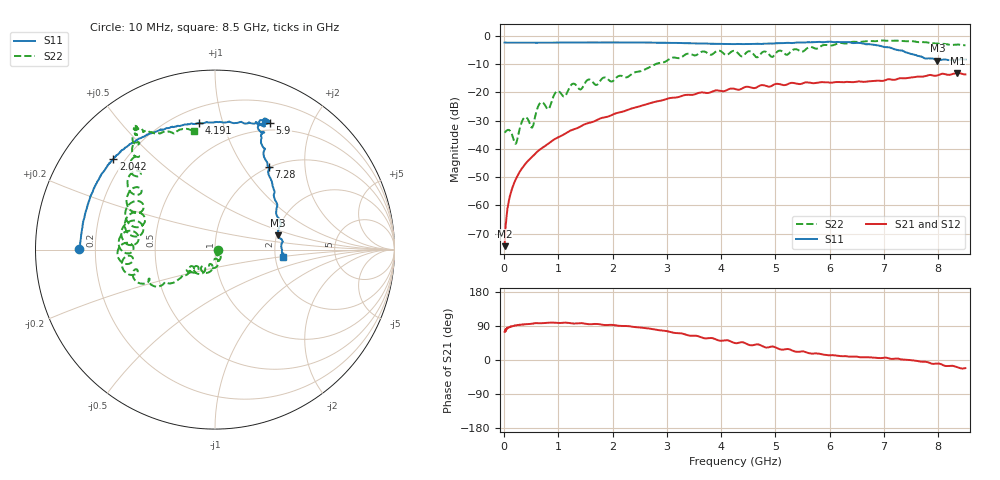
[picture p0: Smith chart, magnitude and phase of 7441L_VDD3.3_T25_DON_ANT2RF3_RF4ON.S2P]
!Agilent Technologies,E5071C,MY46417908,A.11.23
!Date: Mon May 03 19:54:48 2021
!Data & Calibration Information:
!Freq	S11:SOLT2(ON)	S21:SOLT2(ON)	S12:SOLT2(ON)	S22:SOLT2(ON)
!PortZ  Port1:50+j0  Port2:50+j0
!Above PortZ is port z conversion or system Z0 setting when saving the data.
!When reading, reference impedance value at option line is always used.
# Hz S dB R 50
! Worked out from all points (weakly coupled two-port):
!   1601 points, 10 MHz to 8.5 GHz, reference 50 ohm
!   highest |S21| = -13.24 dB at 8.351 GHz (marker M1); lowest = -74.4 dB at 10 MHz (marker M2)
!   lowest |S11| = -8.9 dB at 7.985 GHz (marker M3), VSWR 2.13, Z = 102 + j18.6 ohm
!   |S11| at or under -10 dB: nowhere
!   |S22| runs from -38.2 to -1.7 dB; largest |S21 - S12| = 0.0021
!   S11 on the Smith chart (normalised r, x): 10 MHz: 0.14, +0.00; 2.042 GHz: 0.16, +0.37; 4.191 GHz: 0.29, +0.84; 5.9 GHz: 0.42, +1.44; 7.28 GHz: 0.99, +1.31; 8.5 GHz: 2.19, -0.20
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1e7  -2.43 179.7  -74.42 74.3  -74.75 75.4  -34.26 -2.2
1.16125e8  -2.48 177.2  -56.08 88.4  -56.22 88.7  -33.87 -39.0
2.169438e8  -2.49 174.9  -50.70 91.3  -50.75 91.2  -38.18 -30.7
3.230688e8  -2.50 172.5  -47.10 93.4  -47.13 93.5  -30.69 -31.6
5.194e8  -2.49 168.2  -42.74 96.0  -42.73 96.0  -32.46 -59.8
6.573625e8  -2.50 165.0  -40.29 97.1  -40.31 97.0  -24.00 -66.1
8.218562e8  -2.49 161.4  -38.10 98.4  -38.09 98.5  -25.93 -83.1
9.704312e8  -2.46 158.1  -36.17 97.9  -36.17 97.7  -19.73 -93.5
1.426769e9  -2.42 149.5  -31.91 97.3  -31.92 97.3  -18.81 -118.9
1.554119e9  -2.39 146.8  -30.89 94.5  -30.89 94.5  -15.53 -127.4
2.042294e9  -2.40 138.3  -27.58 91.9  -27.58 91.9  -15.40 -135.8
2.843538e9  -2.49 125.5  -23.16 78.8  -23.17 78.8  -9.75 -145.4
4.191325e9  -2.97 97.2  -18.70 48.0  -18.71 48.0  -5.64 -179.7
4.255e9  -3.00 94.7  -18.85 44.7  -18.85 44.6  -5.44 172.8
4.939506e9  -2.83 76.7  -17.67 35.7  -17.65 35.6  -7.52 159.1
5.671769e9  -2.33 67.4  -16.77 17.0  -16.72 16.8  -4.08 135.7
5.899938e9  -2.28 66.5  -16.49 13.7  -16.43 13.8  -3.31 132.8
7.088538e9  -4.10 63.6  -15.39 4.1  -15.44 4.1  -1.87 123.4
7.279562e9  -5.20 57.1  -15.10 3.0  -15.11 3.0  -1.84 122.6
7.985294e9  -8.85 12.7  -14.07 -9.3  -14.11 -9.1  -2.82 116.4
8.351425e9  -8.50 -3.2  -13.24 -19.1  -13.30 -19.2  -3.14 106.0
8.5e9  -8.45 -5.9  -13.71 -21.4  -13.78 -21.5  -3.45 100.2
